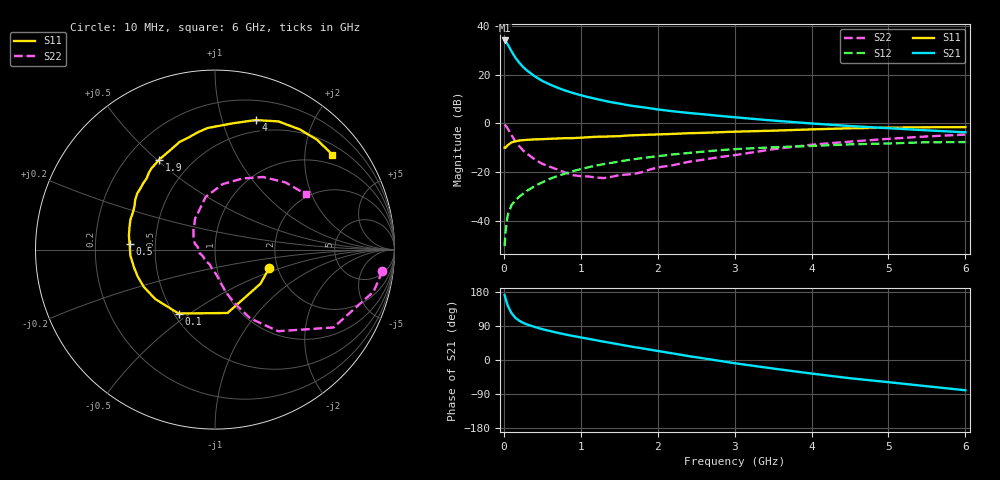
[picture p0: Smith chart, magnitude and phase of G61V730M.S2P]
! SIEMENS Small Signal Semiconductors
! BFG193
! Si NPN RF Bipolar Junction Transistor in SOT223
! VCE = 1.75 V  IC = 30 mA
! Common Emitter S-Parameters:  August  1996
# GHz  S  MA  R  50
!  f  S11  S21  S12  S22
! GHz  MAG  ANG  MAG  ANG  MAG  ANG  MAG  ANG
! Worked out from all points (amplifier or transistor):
!   36 points, 10 MHz to 6 GHz, reference 50 ohm
!   highest |S21| = 33.9 dB at 10 MHz (marker M1)
!   |S21| within 3 dB of that: start of sweep to 74.7 MHz
!   unconditionally stable (mu >= 1): 491.1 MHz to 2.65 GHz
!   at 250 MHz: K = 0.85, MSG = 25.9 dB, |S12| = -28.8 dB
!   at 1.4 GHz: K = 1.05, MAG = 11.0 dB, |S12| = -16.1 dB
!   at 6 GHz: K = 0.93, MSG = 2.0 dB, |S12| = -7.6 dB
!   S11 on the Smith chart (normalised r, x): 10 MHz: 1.80, -0.42; 100 MHz: 0.53, -0.45; 500 MHz: 0.35, +0.03; 1.9 GHz: 0.33, +0.51; 4 GHz: 0.38, +1.29; 6 GHz: 0.73, +2.65
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0.01  0.3189 -19.2  49.71 171.6  0.0031 88.0  0.9408 -7.3
0.02  0.3167 -36.9  48.32 164.2  0.0058 81.9  0.9143 -14.8
0.05  0.36 -78.8  41.36 143.8  0.0133 69.2  0.79 -33.3
0.1  0.41 -119.7  29.83 123.8  0.0215 61.9  0.5748 -52.3
0.15  0.432 -140.4  22.09 111.1  0.0268 60.3  0.4303 -62.9
0.2  0.4477 -152.3  17.48 103.8  0.0317 61.2  0.3435 -68.0
0.25  0.456 -160.7  14.29 98.1  0.0365 61.7  0.2806 -72.5
0.3  0.4618 -167.2  12.1 93.8  0.042 63.0  0.2418 -75.7
0.4  0.4725 -175.9  9.239 87.3  0.0522 63.4  0.1846 -80.8
0.5  0.4772 176.0  7.413 81.3  0.0625 63.1  0.1498 -84.9
0.6  0.486 170.7  6.234 76.5  0.0738 62.6  0.1296 -89.6
0.8  0.5001 160.4  4.686 67.4  0.0949 59.9  0.0989 -103.1
1.1  0.5233 148.2  3.444 55.9  0.1274 55.1  0.0824 -128.6
1.4  0.5451 137.0  2.711 44.8  0.1565 48.7  0.0811 -159.1
1.9  0.59 121.9  2.043 27.3  0.2051 37.8  0.1144 164.5
2.2  0.6109 113.2  1.772 17.3  0.2327 30.5  0.1403 148.6
2.8  0.6616 98.0  1.429 -2.1  0.2837 16.4  0.205 122.9
3.5  0.7111 81.8  1.144 -22.5  0.3258 -1.0  0.2976 100.2
4  0.7563 72.6  1 -35.8  0.3466 -10.8  0.3674 83.3
4.5  0.7968 63.7  0.885 -48.1  0.3741 -20.8  0.425 68.8
5.5  0.8356 47.0  0.723 -69.3  0.4132 -43.6  0.5425 43.6
6  0.841 38.9  0.658 -79.8  0.4159 -56.7  0.5922 31.4
